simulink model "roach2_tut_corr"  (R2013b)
settings: Solver=VariableStepDiscrete  SolverMode=SingleTasking  StartTime=0.0  StopTime=100  RelTol=1e-3
undefined symbols (not defined in the file): add_latency, addr_width, Bit, bitfield, BitWidth, bram_latency, burst_size, casper_library_scopes, conv_latency, data_width, DelayLen, fan_latency, FFTSize, FFTStage, getfield, increment, led, Location, Lower, mult_latency, mux_latency, n_bits, n_bits_data, n_inputs, n_streams, n_taps, neg_latency, negate_latency, nsamples, pfb_size, pulse_len, reset_period, ROACH, ROACH2, snapshot, sx475t, sync_period, sync_period_bits, Upper, UseCounter, Width
libraries: xbsIndex_r4 x24444, casper_library_misc x73, xbsReplacements_r4 x34, casper_library_delays x14, xps_library x7
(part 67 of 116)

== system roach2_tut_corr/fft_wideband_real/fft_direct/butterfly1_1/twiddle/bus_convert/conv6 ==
  note: (ones_bit & 1) -> round-to-even (ones_bit ^ 1) -> round-to-odd (sign_bit & 1)-> round-to-zero (sign_bit ^ 1) -> round-to-inf (X ~| 1) -> round half down (X | 1) -> round half up
  in : Inport
  Concat : xbsIndex_r4/Concat  num_inputs=2  dbl_ovrd=off  block_type=concat
  Constant : xbsIndex_r4/Constant  const=1  gui_display_data_type=Fixed-point  arith_type=Unsigned  n_bits=1  bin_pt=0  preci_type=Single  exp_width=8  frac_width=24  explicit_period=off  period=1  equ=P=C  opselect=C  inp2=PCIN>>17  opr=+  inp1=P  carry=CIN  dbl_ovrd=off  block_type=constant
  Reinterpret : xbsIndex_r4/Reinterpret  force_arith_type=on  arith_type=Unsigned  force_bin_pt=on  bin_pt=0  block_type=reinterpret
  adder : xbsIndex_r4/AddSub  mode=Addition  use_carryin=off  use_carryout=off  en=off  latency=1  precision=User Defined  arith_type="Signed  (2's comp)"  n_bits=19  bin_pt=17  quantization=Truncate  overflow=Wrap  dbl_ovrd=off  use_behavioral_HDL=off  hw_selection=Fabric  pipelined=on  use_rpm=on  block_type=addsub
  almost_half : xbsIndex_r4/Constant  const=131071  gui_display_data_type=Fixed-point  arith_type=Unsigned  n_bits=35  bin_pt=0  preci_type=Single  exp_width=8  frac_width=24  explicit_period=off  period=1  equ=P=C  opselect=C  inp2=PCIN>>17  opr=+  inp1=P  carry=CIN  dbl_ovrd=off  block_type=constant
  bit : xbsIndex_r4/Slice  nbits=1  boolean_output=off  mode=Lower Bit Location + Width  bit1=0  base1=MSB of Input  bit0=17  base0=LSB of Input  dbl_ovrd=off  block_type=slice
  force1 : xbsIndex_r4/Reinterpret  force_arith_type=on  arith_type="Signed  (2's comp)"  force_bin_pt=on  bin_pt=35  block_type=reinterpret
  force2 : xbsIndex_r4/Reinterpret  force_arith_type=off  arith_type="Signed  (2's comp)"  force_bin_pt=on  bin_pt=35  block_type=reinterpret
  tweak_op : xbsIndex_r4/Logical  logical_function=AND  inputs=2  en=off  latency=0  precision=Full  arith_type=Unsigned  n_bits=8  bin_pt=2  align_bp=on  dbl_ovrd=off  block_type=logical
  out : Outport
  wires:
  tweak_op/1 -> Concat/2
  Constant/1 -> tweak_op/2
  bit/1 -> tweak_op/1
  almost_half/1 -> force2/1
  in/1 -> Reinterpret/1, bit/1
  Concat/1 -> force1/1
  Reinterpret/1 -> Concat/1
  force1/1 -> adder/1
  force2/1 -> adder/2
  adder/1 -> out/1

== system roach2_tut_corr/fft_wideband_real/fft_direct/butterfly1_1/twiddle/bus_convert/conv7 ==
  note: (ones_bit & 1) -> round-to-even (ones_bit ^ 1) -> round-to-odd (sign_bit & 1)-> round-to-zero (sign_bit ^ 1) -> round-to-inf (X ~| 1) -> round half down (X | 1) -> round half up
  in : Inport
  Concat : xbsIndex_r4/Concat  num_inputs=2  dbl_ovrd=off  block_type=concat
  Constant : xbsIndex_r4/Constant  const=1  gui_display_data_type=Fixed-point  arith_type=Unsigned  n_bits=1  bin_pt=0  preci_type=Single  exp_width=8  frac_width=24  explicit_period=off  period=1  equ=P=C  opselect=C  inp2=PCIN>>17  opr=+  inp1=P  carry=CIN  dbl_ovrd=off  block_type=constant
  Reinterpret : xbsIndex_r4/Reinterpret  force_arith_type=on  arith_type=Unsigned  force_bin_pt=on  bin_pt=0  block_type=reinterpret
  adder : xbsIndex_r4/AddSub  mode=Addition  use_carryin=off  use_carryout=off  en=off  latency=1  precision=User Defined  arith_type="Signed  (2's comp)"  n_bits=19  bin_pt=17  quantization=Truncate  overflow=Wrap  dbl_ovrd=off  use_behavioral_HDL=off  hw_selection=Fabric  pipelined=on  use_rpm=on  block_type=addsub
  almost_half : xbsIndex_r4/Constant  const=131071  gui_display_data_type=Fixed-point  arith_type=Unsigned  n_bits=35  bin_pt=0  preci_type=Single  exp_width=8  frac_width=24  explicit_period=off  period=1  equ=P=C  opselect=C  inp2=PCIN>>17  opr=+  inp1=P  carry=CIN  dbl_ovrd=off  block_type=constant
  bit : xbsIndex_r4/Slice  nbits=1  boolean_output=off  mode=Lower Bit Location + Width  bit1=0  base1=MSB of Input  bit0=17  base0=LSB of Input  dbl_ovrd=off  block_type=slice
  force1 : xbsIndex_r4/Reinterpret  force_arith_type=on  arith_type="Signed  (2's comp)"  force_bin_pt=on  bin_pt=35  block_type=reinterpret
  force2 : xbsIndex_r4/Reinterpret  force_arith_type=off  arith_type="Signed  (2's comp)"  force_bin_pt=on  bin_pt=35  block_type=reinterpret
  tweak_op : xbsIndex_r4/Logical  logical_function=AND  inputs=2  en=off  latency=0  precision=Full  arith_type=Unsigned  n_bits=8  bin_pt=2  align_bp=on  dbl_ovrd=off  block_type=logical
  out : Outport
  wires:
  tweak_op/1 -> Concat/2
  Constant/1 -> tweak_op/2
  bit/1 -> tweak_op/1
  almost_half/1 -> force2/1
  in/1 -> Reinterpret/1, bit/1
  Concat/1 -> force1/1
  Reinterpret/1 -> Concat/1
  force1/1 -> adder/1
  force2/1 -> adder/2
  adder/1 -> out/1

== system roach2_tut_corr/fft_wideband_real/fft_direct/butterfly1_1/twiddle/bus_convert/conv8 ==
  note: (ones_bit & 1) -> round-to-even (ones_bit ^ 1) -> round-to-odd (sign_bit & 1)-> round-to-zero (sign_bit ^ 1) -> round-to-inf (X ~| 1) -> round half down (X | 1) -> round half up
  in : Inport
  Concat : xbsIndex_r4/Concat  num_inputs=2  dbl_ovrd=off  block_type=concat
  Constant : xbsIndex_r4/Constant  const=1  gui_display_data_type=Fixed-point  arith_type=Unsigned  n_bits=1  bin_pt=0  preci_type=Single  exp_width=8  frac_width=24  explicit_period=off  period=1  equ=P=C  opselect=C  inp2=PCIN>>17  opr=+  inp1=P  carry=CIN  dbl_ovrd=off  block_type=constant
  Reinterpret : xbsIndex_r4/Reinterpret  force_arith_type=on  arith_type=Unsigned  force_bin_pt=on  bin_pt=0  block_type=reinterpret
  adder : xbsIndex_r4/AddSub  mode=Addition  use_carryin=off  use_carryout=off  en=off  latency=1  precision=User Defined  arith_type="Signed  (2's comp)"  n_bits=19  bin_pt=17  quantization=Truncate  overflow=Wrap  dbl_ovrd=off  use_behavioral_HDL=off  hw_selection=Fabric  pipelined=on  use_rpm=on  block_type=addsub
  almost_half : xbsIndex_r4/Constant  const=131071  gui_display_data_type=Fixed-point  arith_type=Unsigned  n_bits=35  bin_pt=0  preci_type=Single  exp_width=8  frac_width=24  explicit_period=off  period=1  equ=P=C  opselect=C  inp2=PCIN>>17  opr=+  inp1=P  carry=CIN  dbl_ovrd=off  block_type=constant
  bit : xbsIndex_r4/Slice  nbits=1  boolean_output=off  mode=Lower Bit Location + Width  bit1=0  base1=MSB of Input  bit0=17  base0=LSB of Input  dbl_ovrd=off  block_type=slice
  force1 : xbsIndex_r4/Reinterpret  force_arith_type=on  arith_type="Signed  (2's comp)"  force_bin_pt=on  bin_pt=35  block_type=reinterpret
  force2 : xbsIndex_r4/Reinterpret  force_arith_type=off  arith_type="Signed  (2's comp)"  force_bin_pt=on  bin_pt=35  block_type=reinterpret
  tweak_op : xbsIndex_r4/Logical  logical_function=AND  inputs=2  en=off  latency=0  precision=Full  arith_type=Unsigned  n_bits=8  bin_pt=2  align_bp=on  dbl_ovrd=off  block_type=logical
  out : Outport
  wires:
  tweak_op/1 -> Concat/2
  Constant/1 -> tweak_op/2
  bit/1 -> tweak_op/1
  almost_half/1 -> force2/1
  in/1 -> Reinterpret/1, bit/1
  Concat/1 -> force1/1
  Reinterpret/1 -> Concat/1
  force1/1 -> adder/1
  force2/1 -> adder/2
  adder/1 -> out/1

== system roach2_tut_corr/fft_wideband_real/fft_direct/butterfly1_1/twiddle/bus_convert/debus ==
  bus_in : Inport
  reinterpret{1..8} (8 alike) : xbsIndex_r4/Reinterpret  force_arith_type=on  arith_type="Signed  (2's comp)"  force_bin_pt=on  bin_pt=34  block_type=reinterpret
  slice1 : xbsIndex_r4/Slice  nbits=37  boolean_output=off  mode=Upper Bit Location + Width  bit1=-259  base1=MSB of Input  bit0=0  base0=LSB of Input  dbl_ovrd=off  block_type=slice
  slice2 : xbsIndex_r4/Slice  nbits=37  boolean_output=off  mode=Upper Bit Location + Width  bit1=-222  base1=MSB of Input  bit0=0  base0=LSB of Input  dbl_ovrd=off  block_type=slice
  slice3 : xbsIndex_r4/Slice  nbits=37  boolean_output=off  mode=Upper Bit Location + Width  bit1=-185  base1=MSB of Input  bit0=0  base0=LSB of Input  dbl_ovrd=off  block_type=slice
  slice4 : xbsIndex_r4/Slice  nbits=37  boolean_output=off  mode=Upper Bit Location + Width  bit1=-148  base1=MSB of Input  bit0=0  base0=LSB of Input  dbl_ovrd=off  block_type=slice
  slice5 : xbsIndex_r4/Slice  nbits=37  boolean_output=off  mode=Upper Bit Location + Width  bit1=-111  base1=MSB of Input  bit0=0  base0=LSB of Input  dbl_ovrd=off  block_type=slice
  slice6 : xbsIndex_r4/Slice  nbits=37  boolean_output=off  mode=Upper Bit Location + Width  bit1=-74  base1=MSB of Input  bit0=0  base0=LSB of Input  dbl_ovrd=off  block_type=slice
  slice7 : xbsIndex_r4/Slice  nbits=37  boolean_output=off  mode=Upper Bit Location + Width  bit1=-37  base1=MSB of Input  bit0=0  base0=LSB of Input  dbl_ovrd=off  block_type=slice
  slice8 : xbsIndex_r4/Slice  nbits=37  boolean_output=off  mode=Upper Bit Location + Width  bit1=0  base1=MSB of Input  bit0=0  base0=LSB of Input  dbl_ovrd=off  block_type=slice
  msb_out8 : Outport
  out7 : Outport  Port=2
  out6 : Outport  Port=3
  out5 : Outport  Port=4
  out4 : Outport  Port=5
  out3 : Outport  Port=6
  out2 : Outport  Port=7
  lsb_out1 : Outport  Port=8
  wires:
  bus_in/1 -> slice8/1, slice7/1, slice6/1, slice5/1, slice4/1, slice3/1, slice2/1, slice1/1
  slice8/1 -> reinterpret8/1
  reinterpret8/1 -> msb_out8/1
  slice7/1 -> reinterpret7/1
  reinterpret7/1 -> out7/1
  slice6/1 -> reinterpret6/1
  reinterpret6/1 -> out6/1
  slice5/1 -> reinterpret5/1
  reinterpret5/1 -> out5/1
  slice4/1 -> reinterpret4/1
  reinterpret4/1 -> out4/1
  slice3/1 -> reinterpret3/1
  reinterpret3/1 -> out3/1
  slice2/1 -> reinterpret2/1
  reinterpret2/1 -> out2/1
  slice1/1 -> reinterpret1/1
  reinterpret1/1 -> lsb_out1/1

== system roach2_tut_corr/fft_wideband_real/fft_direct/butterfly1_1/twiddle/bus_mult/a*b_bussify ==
  in1 : Inport
  in2 : Inport  Port=2
  in3 : Inport  Port=3
  in4 : Inport  Port=4
  concatenate : xbsIndex_r4/Concat  num_inputs=4  dbl_ovrd=off  block_type=concat
  reinterpret{1..4} (4 alike) : xbsIndex_r4/Reinterpret  force_arith_type=on  arith_type=Unsigned  force_bin_pt=on  bin_pt=0  block_type=reinterpret
  bus_out : Outport
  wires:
  concatenate/1 -> bus_out/1
  in1/1 -> reinterpret1/1
  reinterpret1/1 -> concatenate/1
  in2/1 -> reinterpret2/1
  reinterpret2/1 -> concatenate/2
  in3/1 -> reinterpret3/1
  reinterpret3/1 -> concatenate/3
  in4/1 -> reinterpret4/1
  reinterpret4/1 -> concatenate/4

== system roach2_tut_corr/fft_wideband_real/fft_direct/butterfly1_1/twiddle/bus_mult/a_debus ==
  bus_in : Inport
  reinterpret1 : xbsIndex_r4/Reinterpret  force_arith_type=on  arith_type=Unsigned  force_bin_pt=on  bin_pt=0  block_type=reinterpret
  slice1 : xbsIndex_r4/Slice  nbits=36  boolean_output=off  mode=Upper Bit Location + Width  bit1=0  base1=MSB of Input  bit0=0  base0=LSB of Input  dbl_ovrd=off  block_type=slice
  msb_lsb_out1 : Outport
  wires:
  bus_in/1 -> slice1/1
  slice1/1 -> reinterpret1/1
  reinterpret1/1 -> msb_lsb_out1/1

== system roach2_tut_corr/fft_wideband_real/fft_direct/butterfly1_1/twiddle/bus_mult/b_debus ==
  bus_in : Inport
  reinterpret{1..4} (4 alike) : xbsIndex_r4/Reinterpret  force_arith_type=on  arith_type=Unsigned  force_bin_pt=on  bin_pt=0  block_type=reinterpret
  slice1 : xbsIndex_r4/Slice  nbits=36  boolean_output=off  mode=Upper Bit Location + Width  bit1=-108  base1=MSB of Input  bit0=0  base0=LSB of Input  dbl_ovrd=off  block_type=slice
  slice2 : xbsIndex_r4/Slice  nbits=36  boolean_output=off  mode=Upper Bit Location + Width  bit1=-72  base1=MSB of Input  bit0=0  base0=LSB of Input  dbl_ovrd=off  block_type=slice
  slice3 : xbsIndex_r4/Slice  nbits=36  boolean_output=off  mode=Upper Bit Location + Width  bit1=-36  base1=MSB of Input  bit0=0  base0=LSB of Input  dbl_ovrd=off  block_type=slice
  slice4 : xbsIndex_r4/Slice  nbits=36  boolean_output=off  mode=Upper Bit Location + Width  bit1=0  base1=MSB of Input  bit0=0  base0=LSB of Input  dbl_ovrd=off  block_type=slice
  msb_out4 : Outport
  out3 : Outport  Port=2
  out2 : Outport  Port=3
  lsb_out1 : Outport  Port=4
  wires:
  bus_in/1 -> slice4/1, slice3/1, slice2/1, slice1/1
  slice4/1 -> reinterpret4/1
  reinterpret4/1 -> msb_out4/1
  slice3/1 -> reinterpret3/1
  reinterpret3/1 -> out3/1
  slice2/1 -> reinterpret2/1
  reinterpret2/1 -> out2/1
  slice1/1 -> reinterpret1/1
  reinterpret1/1 -> lsb_out1/1

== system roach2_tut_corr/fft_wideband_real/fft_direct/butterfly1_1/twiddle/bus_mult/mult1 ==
  a : Inport
  b : Inport  Port=2
  a_expand : Subsystem  AncestorBlock=casper_library_flow_control/bus_expand
  a_replicate : Subsystem  AncestorBlock=casper_library_bus/bus_replicate
  addsub_im : xbsIndex_r4/AddSub  mode=Addition  use_carryin=off  use_carryout=off  en=off  latency=1  precision=Full  arith_type=Unsigned  n_bits=16  bin_pt=14  quantization=Truncate  overflow=Wrap  dbl_ovrd=off  use_behavioral_HDL=on  hw_selection=Fabric  pipelined=on  use_rpm=on  block_type=addsub
  addsub_re : xbsIndex_r4/AddSub  mode=Subtraction  use_carryin=off  use_carryout=off  en=off  latency=1  precision=Full  arith_type=Unsigned  n_bits=16  bin_pt=14  quantization=Truncate  overflow=Wrap  dbl_ovrd=off  use_behavioral_HDL=on  hw_selection=Fabric  pipelined=on  use_rpm=on  block_type=addsub
  b_expand : Subsystem  AncestorBlock=casper_library_flow_control/bus_expand
  b_replicate : Subsystem  AncestorBlock=casper_library_bus/bus_replicate
  convert_im : xbsIndex_r4/Convert  gui_display_data_type=Fixed-point  arith_type="Signed  (2's comp)"  n_bits=37  bin_pt=34  float_type=Single  exp_bits=8  fraction_bits=24  quantization=Truncate  overflow=Wrap  en=off  latency=0  dbl_ovrd=off  pipeline=on  block_type=convert
  convert_re : xbsIndex_r4/Convert  gui_display_data_type=Fixed-point  arith_type="Signed  (2's comp)"  n_bits=37  bin_pt=34  float_type=Single  exp_bits=8  fraction_bits=24  quantization=Truncate  overflow=Wrap  en=off  latency=0  dbl_ovrd=off  pipeline=on  block_type=convert
  imim : xbsIndex_r4/Mult  precision=Full  arith_type="Signed  (2's comp)"  n_bits=16  bin_pt=14  quantization=Truncate  overflow=Wrap  en=off  latency=3  dbl_ovrd=off  use_behavioral_HDL=on  opt=Speed  use_embedded=off  optimum_pipeline=off  pipeline=on  use_rpm=on  placement_style=Triangular  block_type=mult
  imre : xbsIndex_r4/Mult  precision=Full  arith_type="Signed  (2's comp)"  n_bits=16  bin_pt=14  quantization=Truncate  overflow=Wrap  en=off  latency=3  dbl_ovrd=off  use_behavioral_HDL=on  opt=Speed  use_embedded=off  optimum_pipeline=off  pipeline=on  use_rpm=on  placement_style=Triangular  block_type=mult
  reim : xbsIndex_r4/Mult  precision=Full  arith_type="Signed  (2's comp)"  n_bits=16  bin_pt=14  quantization=Truncate  overflow=Wrap  en=off  latency=3  dbl_ovrd=off  use_behavioral_HDL=on  opt=Speed  use_embedded=off  optimum_pipeline=off  pipeline=on  use_rpm=on  placement_style=Triangular  block_type=mult
  rere : xbsIndex_r4/Mult  precision=Full  arith_type="Signed  (2's comp)"  n_bits=16  bin_pt=14  quantization=Truncate  overflow=Wrap  en=off  latency=3  dbl_ovrd=off  use_behavioral_HDL=on  opt=Speed  use_embedded=off  optimum_pipeline=off  pipeline=on  use_rpm=on  placement_style=Triangular  block_type=mult
  ri_to_c : casper_library_misc/ri_to_c
  ab : Outport
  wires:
  a/1 -> a_replicate/1(in)
  b/1 -> b_replicate/1(in)
  a_replicate/1(out) -> a_expand/1(bus_in)
  b_replicate/1(out) -> b_expand/1(bus_in)
  a_expand/1(msb_out4) -> rere/1
  b_expand/1(msb_out4) -> rere/2
  a_expand/2(out3) -> imim/1
  b_expand/2(out3) -> imim/2
  a_expand/4(lsb_out1) -> imre/1
  b_expand/3(out2) -> imre/2
  a_expand/3(out2) -> reim/1
  b_expand/4(lsb_out1) -> reim/2
  rere/1 -> addsub_re/1
  imim/1 -> addsub_re/2
  imre/1 -> addsub_im/1
  reim/1 -> addsub_im/2
  addsub_re/1 -> convert_re/1
  addsub_im/1 -> convert_im/1
  convert_re/1 -> ri_to_c/1
  convert_im/1 -> ri_to_c/2
  ri_to_c/1 -> ab/1

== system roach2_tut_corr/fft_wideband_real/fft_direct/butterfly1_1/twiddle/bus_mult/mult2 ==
  a : Inport
  b : Inport  Port=2
  a_expand : Subsystem  AncestorBlock=casper_library_flow_control/bus_expand
  a_replicate : Subsystem  AncestorBlock=casper_library_bus/bus_replicate
  addsub_im : xbsIndex_r4/AddSub  mode=Addition  use_carryin=off  use_carryout=off  en=off  latency=1  precision=Full  arith_type=Unsigned  n_bits=16  bin_pt=14  quantization=Truncate  overflow=Wrap  dbl_ovrd=off  use_behavioral_HDL=on  hw_selection=Fabric  pipelined=on  use_rpm=on  block_type=addsub
  addsub_re : xbsIndex_r4/AddSub  mode=Subtraction  use_carryin=off  use_carryout=off  en=off  latency=1  precision=Full  arith_type=Unsigned  n_bits=16  bin_pt=14  quantization=Truncate  overflow=Wrap  dbl_ovrd=off  use_behavioral_HDL=on  hw_selection=Fabric  pipelined=on  use_rpm=on  block_type=addsub
  b_expand : Subsystem  AncestorBlock=casper_library_flow_control/bus_expand
  b_replicate : Subsystem  AncestorBlock=casper_library_bus/bus_replicate
  convert_im : xbsIndex_r4/Convert  gui_display_data_type=Fixed-point  arith_type="Signed  (2's comp)"  n_bits=37  bin_pt=34  float_type=Single  exp_bits=8  fraction_bits=24  quantization=Truncate  overflow=Wrap  en=off  latency=0  dbl_ovrd=off  pipeline=on  block_type=convert
  convert_re : xbsIndex_r4/Convert  gui_display_data_type=Fixed-point  arith_type="Signed  (2's comp)"  n_bits=37  bin_pt=34  float_type=Single  exp_bits=8  fraction_bits=24  quantization=Truncate  overflow=Wrap  en=off  latency=0  dbl_ovrd=off  pipeline=on  block_type=convert
  imim : xbsIndex_r4/Mult  precision=Full  arith_type="Signed  (2's comp)"  n_bits=16  bin_pt=14  quantization=Truncate  overflow=Wrap  en=off  latency=3  dbl_ovrd=off  use_behavioral_HDL=on  opt=Speed  use_embedded=off  optimum_pipeline=off  pipeline=on  use_rpm=on  placement_style=Triangular  block_type=mult
  imre : xbsIndex_r4/Mult  precision=Full  arith_type="Signed  (2's comp)"  n_bits=16  bin_pt=14  quantization=Truncate  overflow=Wrap  en=off  latency=3  dbl_ovrd=off  use_behavioral_HDL=on  opt=Speed  use_embedded=off  optimum_pipeline=off  pipeline=on  use_rpm=on  placement_style=Triangular  block_type=mult
  reim : xbsIndex_r4/Mult  precision=Full  arith_type="Signed  (2's comp)"  n_bits=16  bin_pt=14  quantization=Truncate  overflow=Wrap  en=off  latency=3  dbl_ovrd=off  use_behavioral_HDL=on  opt=Speed  use_embedded=off  optimum_pipeline=off  pipeline=on  use_rpm=on  placement_style=Triangular  block_type=mult
  rere : xbsIndex_r4/Mult  precision=Full  arith_type="Signed  (2's comp)"  n_bits=16  bin_pt=14  quantization=Truncate  overflow=Wrap  en=off  latency=3  dbl_ovrd=off  use_behavioral_HDL=on  opt=Speed  use_embedded=off  optimum_pipeline=off  pipeline=on  use_rpm=on  placement_style=Triangular  block_type=mult
  ri_to_c : casper_library_misc/ri_to_c
  ab : Outport
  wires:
  a/1 -> a_replicate/1(in)
  b/1 -> b_replicate/1(in)
  a_replicate/1(out) -> a_expand/1(bus_in)
  b_replicate/1(out) -> b_expand/1(bus_in)
  a_expand/1(msb_out4) -> rere/1
  b_expand/1(msb_out4) -> rere/2
  a_expand/2(out3) -> imim/1
  b_expand/2(out3) -> imim/2
  a_expand/4(lsb_out1) -> imre/1
  b_expand/3(out2) -> imre/2
  a_expand/3(out2) -> reim/1
  b_expand/4(lsb_out1) -> reim/2
  rere/1 -> addsub_re/1
  imim/1 -> addsub_re/2
  imre/1 -> addsub_im/1
  reim/1 -> addsub_im/2
  addsub_re/1 -> convert_re/1
  addsub_im/1 -> convert_im/1
  convert_re/1 -> ri_to_c/1
  convert_im/1 -> ri_to_c/2
  ri_to_c/1 -> ab/1

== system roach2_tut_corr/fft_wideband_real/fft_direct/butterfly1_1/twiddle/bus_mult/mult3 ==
  a : Inport
  b : Inport  Port=2
  a_expand : Subsystem  AncestorBlock=casper_library_flow_control/bus_expand
  a_replicate : Subsystem  AncestorBlock=casper_library_bus/bus_replicate
  addsub_im : xbsIndex_r4/AddSub  mode=Addition  use_carryin=off  use_carryout=off  en=off  latency=1  precision=Full  arith_type=Unsigned  n_bits=16  bin_pt=14  quantization=Truncate  overflow=Wrap  dbl_ovrd=off  use_behavioral_HDL=on  hw_selection=Fabric  pipelined=on  use_rpm=on  block_type=addsub
  addsub_re : xbsIndex_r4/AddSub  mode=Subtraction  use_carryin=off  use_carryout=off  en=off  latency=1  precision=Full  arith_type=Unsigned  n_bits=16  bin_pt=14  quantization=Truncate  overflow=Wrap  dbl_ovrd=off  use_behavioral_HDL=on  hw_selection=Fabric  pipelined=on  use_rpm=on  block_type=addsub
  b_expand : Subsystem  AncestorBlock=casper_library_flow_control/bus_expand
  b_replicate : Subsystem  AncestorBlock=casper_library_bus/bus_replicate
  convert_im : xbsIndex_r4/Convert  gui_display_data_type=Fixed-point  arith_type="Signed  (2's comp)"  n_bits=37  bin_pt=34  float_type=Single  exp_bits=8  fraction_bits=24  quantization=Truncate  overflow=Wrap  en=off  latency=0  dbl_ovrd=off  pipeline=on  block_type=convert
  convert_re : xbsIndex_r4/Convert  gui_display_data_type=Fixed-point  arith_type="Signed  (2's comp)"  n_bits=37  bin_pt=34  float_type=Single  exp_bits=8  fraction_bits=24  quantization=Truncate  overflow=Wrap  en=off  latency=0  dbl_ovrd=off  pipeline=on  block_type=convert
  imim : xbsIndex_r4/Mult  precision=Full  arith_type="Signed  (2's comp)"  n_bits=16  bin_pt=14  quantization=Truncate  overflow=Wrap  en=off  latency=3  dbl_ovrd=off  use_behavioral_HDL=on  opt=Speed  use_embedded=off  optimum_pipeline=off  pipeline=on  use_rpm=on  placement_style=Triangular  block_type=mult
  imre : xbsIndex_r4/Mult  precision=Full  arith_type="Signed  (2's comp)"  n_bits=16  bin_pt=14  quantization=Truncate  overflow=Wrap  en=off  latency=3  dbl_ovrd=off  use_behavioral_HDL=on  opt=Speed  use_embedded=off  optimum_pipeline=off  pipeline=on  use_rpm=on  placement_style=Triangular  block_type=mult
  reim : xbsIndex_r4/Mult  precision=Full  arith_type="Signed  (2's comp)"  n_bits=16  bin_pt=14  quantization=Truncate  overflow=Wrap  en=off  latency=3  dbl_ovrd=off  use_behavioral_HDL=on  opt=Speed  use_embedded=off  optimum_pipeline=off  pipeline=on  use_rpm=on  placement_style=Triangular  block_type=mult
  rere : xbsIndex_r4/Mult  precision=Full  arith_type="Signed  (2's comp)"  n_bits=16  bin_pt=14  quantization=Truncate  overflow=Wrap  en=off  latency=3  dbl_ovrd=off  use_behavioral_HDL=on  opt=Speed  use_embedded=off  optimum_pipeline=off  pipeline=on  use_rpm=on  placement_style=Triangular  block_type=mult
  ri_to_c : casper_library_misc/ri_to_c
  ab : Outport
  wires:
  a/1 -> a_replicate/1(in)
  b/1 -> b_replicate/1(in)
  a_replicate/1(out) -> a_expand/1(bus_in)
  b_replicate/1(out) -> b_expand/1(bus_in)
  a_expand/1(msb_out4) -> rere/1
  b_expand/1(msb_out4) -> rere/2
  a_expand/2(out3) -> imim/1
  b_expand/2(out3) -> imim/2
  a_expand/4(lsb_out1) -> imre/1
  b_expand/3(out2) -> imre/2
  a_expand/3(out2) -> reim/1
  b_expand/4(lsb_out1) -> reim/2
  rere/1 -> addsub_re/1
  imim/1 -> addsub_re/2
  imre/1 -> addsub_im/1
  reim/1 -> addsub_im/2
  addsub_re/1 -> convert_re/1
  addsub_im/1 -> convert_im/1
  convert_re/1 -> ri_to_c/1
  convert_im/1 -> ri_to_c/2
  ri_to_c/1 -> ab/1

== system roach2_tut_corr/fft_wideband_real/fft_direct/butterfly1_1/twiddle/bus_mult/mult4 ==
  a : Inport
  b : Inport  Port=2
  a_expand : Subsystem  AncestorBlock=casper_library_flow_control/bus_expand
  a_replicate : Subsystem  AncestorBlock=casper_library_bus/bus_replicate
  addsub_im : xbsIndex_r4/AddSub  mode=Addition  use_carryin=off  use_carryout=off  en=off  latency=1  precision=Full  arith_type=Unsigned  n_bits=16  bin_pt=14  quantization=Truncate  overflow=Wrap  dbl_ovrd=off  use_behavioral_HDL=on  hw_selection=Fabric  pipelined=on  use_rpm=on  block_type=addsub
  addsub_re : xbsIndex_r4/AddSub  mode=Subtraction  use_carryin=off  use_carryout=off  en=off  latency=1  precision=Full  arith_type=Unsigned  n_bits=16  bin_pt=14  quantization=Truncate  overflow=Wrap  dbl_ovrd=off  use_behavioral_HDL=on  hw_selection=Fabric  pipelined=on  use_rpm=on  block_type=addsub
  b_expand : Subsystem  AncestorBlock=casper_library_flow_control/bus_expand
  b_replicate : Subsystem  AncestorBlock=casper_library_bus/bus_replicate
  convert_im : xbsIndex_r4/Convert  gui_display_data_type=Fixed-point  arith_type="Signed  (2's comp)"  n_bits=37  bin_pt=34  float_type=Single  exp_bits=8  fraction_bits=24  quantization=Truncate  overflow=Wrap  en=off  latency=0  dbl_ovrd=off  pipeline=on  block_type=convert
  convert_re : xbsIndex_r4/Convert  gui_display_data_type=Fixed-point  arith_type="Signed  (2's comp)"  n_bits=37  bin_pt=34  float_type=Single  exp_bits=8  fraction_bits=24  quantization=Truncate  overflow=Wrap  en=off  latency=0  dbl_ovrd=off  pipeline=on  block_type=convert
  imim : xbsIndex_r4/Mult  precision=Full  arith_type="Signed  (2's comp)"  n_bits=16  bin_pt=14  quantization=Truncate  overflow=Wrap  en=off  latency=3  dbl_ovrd=off  use_behavioral_HDL=on  opt=Speed  use_embedded=off  optimum_pipeline=off  pipeline=on  use_rpm=on  placement_style=Triangular  block_type=mult
  imre : xbsIndex_r4/Mult  precision=Full  arith_type="Signed  (2's comp)"  n_bits=16  bin_pt=14  quantization=Truncate  overflow=Wrap  en=off  latency=3  dbl_ovrd=off  use_behavioral_HDL=on  opt=Speed  use_embedded=off  optimum_pipeline=off  pipeline=on  use_rpm=on  placement_style=Triangular  block_type=mult
  reim : xbsIndex_r4/Mult  precision=Full  arith_type="Signed  (2's comp)"  n_bits=16  bin_pt=14  quantization=Truncate  overflow=Wrap  en=off  latency=3  dbl_ovrd=off  use_behavioral_HDL=on  opt=Speed  use_embedded=off  optimum_pipeline=off  pipeline=on  use_rpm=on  placement_style=Triangular  block_type=mult
  rere : xbsIndex_r4/Mult  precision=Full  arith_type="Signed  (2's comp)"  n_bits=16  bin_pt=14  quantization=Truncate  overflow=Wrap  en=off  latency=3  dbl_ovrd=off  use_behavioral_HDL=on  opt=Speed  use_embedded=off  optimum_pipeline=off  pipeline=on  use_rpm=on  placement_style=Triangular  block_type=mult
  ri_to_c : casper_library_misc/ri_to_c
  ab : Outport
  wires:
  a/1 -> a_replicate/1(in)
  b/1 -> b_replicate/1(in)
  a_replicate/1(out) -> a_expand/1(bus_in)
  b_replicate/1(out) -> b_expand/1(bus_in)
  a_expand/1(msb_out4) -> rere/1
  b_expand/1(msb_out4) -> rere/2
  a_expand/2(out3) -> imim/1
  b_expand/2(out3) -> imim/2
  a_expand/4(lsb_out1) -> imre/1
  b_expand/3(out2) -> imre/2
  a_expand/3(out2) -> reim/1
  b_expand/4(lsb_out1) -> reim/2
  rere/1 -> addsub_re/1
  imim/1 -> addsub_re/2
  imre/1 -> addsub_im/1
  reim/1 -> addsub_im/2
  addsub_re/1 -> convert_re/1
  addsub_im/1 -> convert_im/1
  convert_re/1 -> ri_to_c/1
  convert_im/1 -> ri_to_c/2
  ri_to_c/1 -> ab/1

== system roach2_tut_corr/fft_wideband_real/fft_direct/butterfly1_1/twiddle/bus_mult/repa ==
  in : Inport
  bussify : Subsystem  AncestorBlock=casper_library_flow_control/bus_create
  din0_0 : xbsIndex_r4/Delay  rst=off  infoeditControl=Selection of Reset will increase slice count due to use of real FFs and instead of SRLs  en=off  latency=1  dbl_ovrd=off  reg_retiming=on  block_type=delay
  din1_0 : xbsIndex_r4/Delay  rst=off  infoeditControl=Selection of Reset will increase slice count due to use of real FFs and instead of SRLs  en=off  latency=1  dbl_ovrd=off  reg_retiming=off  block_type=delay
  out : Outport
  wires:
  in/1 -> din0_0/1
  din0_0/1 -> din1_0/1
  din1_0/1 -> bussify/1(in1)
  bussify/1(bus_out) -> out/1

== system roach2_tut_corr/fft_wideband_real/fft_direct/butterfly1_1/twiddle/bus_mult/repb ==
  in : Inport
  bussify : Subsystem  AncestorBlock=casper_library_flow_control/bus_create
  din0_0 : xbsIndex_r4/Delay  rst=off  infoeditControl=Selection of Reset will increase slice count due to use of real FFs and instead of SRLs  en=off  latency=1  dbl_ovrd=off  reg_retiming=on  block_type=delay
  din1_0 : xbsIndex_r4/Delay  rst=off  infoeditControl=Selection of Reset will increase slice count due to use of real FFs and instead of SRLs  en=off  latency=1  dbl_ovrd=off  reg_retiming=off  block_type=delay
  out : Outport
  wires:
  in/1 -> din0_0/1
  din0_0/1 -> din1_0/1
  din1_0/1 -> bussify/1(in1)
  bussify/1(bus_out) -> out/1

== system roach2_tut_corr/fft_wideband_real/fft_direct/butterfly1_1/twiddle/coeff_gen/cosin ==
  theta : Inport
  misci : Inport  Port=2
  Constant4 : xbsIndex_r4/Constant  const=0  gui_display_data_type=Fixed-point  arith_type=Unsigned  n_bits=1  bin_pt=0  preci_type=Single  exp_width=8  frac_width=24  explicit_period=on  period=1  equ=P=C  opselect=C  inp2=PCIN>>17  opr=+  inp1=P  carry=CIN  dbl_ovrd=off  block_type=constant
  Constant5 : xbsIndex_r4/Constant  const=0  gui_display_data_type=Fixed-point  arith_type=Unsigned  n_bits=1  bin_pt=0  preci_type=Single  exp_width=8  frac_width=24  explicit_period=on  period=1  equ=P=C  opselect=C  inp2=PCIN>>17  opr=+  inp1=P  carry=CIN  dbl_ovrd=off  block_type=constant
  Delay : xbsIndex_r4/Delay  rst=off  infoeditControl=Selection of Reset will increase slice count due to use of real FFs and instead of SRLs  en=off  latency=bram_latency  dbl_ovrd=off  reg_retiming=on  block_type=delay
  Delay10 : xbsIndex_r4/Delay  rst=off  infoeditControl=Selection of Reset will increase slice count due to use of real FFs and instead of SRLs  en=off  latency=bram_latency  dbl_ovrd=off  reg_retiming=on  block_type=delay
  Delay8 : xbsIndex_r4/Delay  rst=off  infoeditControl=Selection of Reset will increase slice count due to use of real FFs and instead of SRLs  en=off  latency=bram_latency  dbl_ovrd=off  reg_retiming=on  block_type=delay
  ROM : xbsIndex_r4/ROM  depth=2^(9)  initVector=[131072 68614225921 68508844034 68403462150 68298080266 68192436239 68087054358 67981672478 67876290599 67770908722 67665526846 67560144971 67455025241 67349643368 67244261497 67138879627 67033759902 66928378034 66822996168 66717876447 66612756727 66507374864 66402255146 66297135430 66192015715 66086896001 65981776289 65876656577 65771536867 65666679302 65561559595 65456702032 65351844471 65246986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  distributed_mem=Block RAM  rst=off  init_reg=0  en=off  latency=bram_latency  gui_display_data_type=Fixed-point  arith_type=Unsigned  n_bits=n_bits*2  bin_pt=0  preci_type=Single  exp_width=8  frac_width=24  dbl_ovrd=off  optimize=Speed  use_rpm=on  block_type=sprom
  Terminator : Terminator
  Terminator1 : Terminator
  Terminator4 : Terminator
  add_convert0 : Subsystem
  add_convert1 : Subsystem
  assert : xbsIndex_r4/Assert  assert_type=on  type_source=Explicitly  gui_display_data_type=Fixed-point  arith_type=Unsigned  n_bits=9  bin_pt=0  preci_type=Single  exp_width=8  frac_width=24  assert_rate=off  rate_source=Explicitly  period=1  output_port=on  block_type=assert
  c_to_ri : casper_library_misc/c_to_ri  n_bits=n_bits  bin_pt=bin_pt
  invert0 : Subsystem
  invert1 : Subsystem
  -sin : Outport
  -cos : Outport  Port=2
  misco : Outport  Port=3
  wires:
  theta/1 -> assert/1
  assert/1 -> add_convert0/1(theta), add_convert1/1(theta)
  Constant4/1 -> add_convert0/2(misci)
  add_convert0/3(misco) -> Terminator/1
  misci/1 -> add_convert1/2(misci)
  add_convert1/3(misco) -> Delay/1
  add_convert0/2(add) -> ROM/1
  add_convert1/2(add) -> Terminator4/1
  ROM/1 -> c_to_ri/1
  add_convert1/1(negate) -> Delay8/1
  add_convert0/1(negate) -> Delay10/1
  Delay10/1 -> invert0/1(negate)
  Constant5/1 -> invert0/3(misci)
  c_to_ri/1 -> invert0/2(in)
  Delay8/1 -> invert1/1(negate)
  c_to_ri/2 -> invert1/2(in)
  invert0/2(misco) -> Terminator1/1
  Delay/1 -> invert1/3(misci)
  invert0/1(out) -> -sin/1
  invert1/1(out) -> -cos/1
  invert1/2(misco) -> misco/1

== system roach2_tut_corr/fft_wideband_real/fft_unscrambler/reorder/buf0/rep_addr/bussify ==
  in1 : Inport
  in2 : Inport  Port=2
  in3 : Inport  Port=3
  in4 : Inport  Port=4
  concatenate : xbsIndex_r4/Concat  num_inputs=4  dbl_ovrd=off  block_type=concat
  reinterpret{1..4} (4 alike) : xbsIndex_r4/Reinterpret  force_arith_type=on  arith_type=Unsigned  force_bin_pt=on  bin_pt=0  block_type=reinterpret
  bus_out : Outport
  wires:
  concatenate/1 -> bus_out/1
  in1/1 -> reinterpret1/1
  reinterpret1/1 -> concatenate/1
  in2/1 -> reinterpret2/1
  reinterpret2/1 -> concatenate/2
  in3/1 -> reinterpret3/1
  reinterpret3/1 -> concatenate/3
  in4/1 -> reinterpret4/1
  reinterpret4/1 -> concatenate/4

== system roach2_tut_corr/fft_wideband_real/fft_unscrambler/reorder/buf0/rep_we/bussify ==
  in1 : Inport
  in2 : Inport  Port=2
  in3 : Inport  Port=3
  in4 : Inport  Port=4
  concatenate : xbsIndex_r4/Concat  num_inputs=4  dbl_ovrd=off  block_type=concat
  reinterpret{1..4} (4 alike) : xbsIndex_r4/Reinterpret  force_arith_type=on  arith_type=Unsigned  force_bin_pt=on  bin_pt=0  block_type=reinterpret
  bus_out : Outport
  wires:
  concatenate/1 -> bus_out/1
  in1/1 -> reinterpret1/1
  reinterpret1/1 -> concatenate/1
  in2/1 -> reinterpret2/1
  reinterpret2/1 -> concatenate/2
  in3/1 -> reinterpret3/1
  reinterpret3/1 -> concatenate/3
  in4/1 -> reinterpret4/1
  reinterpret4/1 -> concatenate/4

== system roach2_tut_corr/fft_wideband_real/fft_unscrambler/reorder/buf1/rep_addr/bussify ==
  in1 : Inport
  in2 : Inport  Port=2
  in3 : Inport  Port=3
  in4 : Inport  Port=4
  concatenate : xbsIndex_r4/Concat  num_inputs=4  dbl_ovrd=off  block_type=concat
  reinterpret{1..4} (4 alike) : xbsIndex_r4/Reinterpret  force_arith_type=on  arith_type=Unsigned  force_bin_pt=on  bin_pt=0  block_type=reinterpret
  bus_out : Outport
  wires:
  concatenate/1 -> bus_out/1
  in1/1 -> reinterpret1/1
  reinterpret1/1 -> concatenate/1
  in2/1 -> reinterpret2/1
  reinterpret2/1 -> concatenate/2
  in3/1 -> reinterpret3/1
  reinterpret3/1 -> concatenate/3
  in4/1 -> reinterpret4/1
  reinterpret4/1 -> concatenate/4

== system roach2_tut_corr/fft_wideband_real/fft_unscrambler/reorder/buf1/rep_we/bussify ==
  in1 : Inport
  in2 : Inport  Port=2
  in3 : Inport  Port=3
  in4 : Inport  Port=4
  concatenate : xbsIndex_r4/Concat  num_inputs=4  dbl_ovrd=off  block_type=concat
  reinterpret{1..4} (4 alike) : xbsIndex_r4/Reinterpret  force_arith_type=on  arith_type=Unsigned  force_bin_pt=on  bin_pt=0  block_type=reinterpret
  bus_out : Outport
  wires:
  concatenate/1 -> bus_out/1
  in1/1 -> reinterpret1/1
  reinterpret1/1 -> concatenate/1
  in2/1 -> reinterpret2/1
  reinterpret2/1 -> concatenate/2
  in3/1 -> reinterpret3/1
  reinterpret3/1 -> concatenate/3
  in4/1 -> reinterpret4/1
  reinterpret4/1 -> concatenate/4

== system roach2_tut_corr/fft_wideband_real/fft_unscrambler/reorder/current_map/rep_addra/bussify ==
  in1 : Inport
  reinterpret1 : xbsIndex_r4/Reinterpret  force_arith_type=on  arith_type=Unsigned  force_bin_pt=on  bin_pt=0  block_type=reinterpret
  bus_out : Outport
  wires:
  in1/1 -> reinterpret1/1
  reinterpret1/1 -> bus_out/1

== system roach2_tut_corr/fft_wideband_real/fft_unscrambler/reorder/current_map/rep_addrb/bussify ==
  in1 : Inport
  reinterpret1 : xbsIndex_r4/Reinterpret  force_arith_type=on  arith_type=Unsigned  force_bin_pt=on  bin_pt=0  block_type=reinterpret
  bus_out : Outport
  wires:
  in1/1 -> reinterpret1/1
  reinterpret1/1 -> bus_out/1

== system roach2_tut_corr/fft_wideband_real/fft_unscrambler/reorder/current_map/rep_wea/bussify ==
  in1 : Inport
  reinterpret1 : xbsIndex_r4/Reinterpret  force_arith_type=on  arith_type=Unsigned  force_bin_pt=on  bin_pt=0  block_type=reinterpret
  bus_out : Outport
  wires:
  in1/1 -> reinterpret1/1
  reinterpret1/1 -> bus_out/1

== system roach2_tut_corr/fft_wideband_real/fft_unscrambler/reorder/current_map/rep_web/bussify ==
  in1 : Inport
  reinterpret1 : xbsIndex_r4/Reinterpret  force_arith_type=on  arith_type=Unsigned  force_bin_pt=on  bin_pt=0  block_type=reinterpret
  bus_out : Outport
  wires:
  in1/1 -> reinterpret1/1
  reinterpret1/1 -> bus_out/1

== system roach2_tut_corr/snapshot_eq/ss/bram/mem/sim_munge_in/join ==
  in1 : Inport
  in2 : Inport  Port=2
  concatenate : xbsIndex_r4/Concat  num_inputs=2  dbl_ovrd=off  block_type=concat
  reinterpret1 : xbsIndex_r4/Reinterpret  force_arith_type=on  arith_type=Unsigned  force_bin_pt=on  bin_pt=0  block_type=reinterpret
  reinterpret2 : xbsIndex_r4/Reinterpret  force_arith_type=on  arith_type=Unsigned  force_bin_pt=on  bin_pt=0  block_type=reinterpret
  bus_out : Outport
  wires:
  concatenate/1 -> bus_out/1
  in1/1 -> reinterpret1/1
  reinterpret1/1 -> concatenate/1
  in2/1 -> reinterpret2/1
  reinterpret2/1 -> concatenate/2

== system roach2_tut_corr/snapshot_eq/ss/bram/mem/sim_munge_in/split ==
  bus_in : Inport
  reinterpret1 : xbsIndex_r4/Reinterpret  force_arith_type=on  arith_type=Unsigned  force_bin_pt=on  bin_pt=0  block_type=reinterpret
  reinterpret2 : xbsIndex_r4/Reinterpret  force_arith_type=on  arith_type=Unsigned  force_bin_pt=on  bin_pt=0  block_type=reinterpret
  slice1 : xbsIndex_r4/Slice  nbits=32  boolean_output=off  mode=Upper Bit Location + Width  bit1=-32  base1=MSB of Input  bit0=0  base0=LSB of Input  dbl_ovrd=off  block_type=slice
  slice2 : xbsIndex_r4/Slice  nbits=32  boolean_output=off  mode=Upper Bit Location + Width  bit1=0  base1=MSB of Input  bit0=0  base0=LSB of Input  dbl_ovrd=off  block_type=slice
  msb_out2 : Outport
  lsb_out1 : Outport  Port=2
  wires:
  bus_in/1 -> slice2/1, slice1/1
  slice2/1 -> reinterpret2/1
  reinterpret2/1 -> msb_out2/1
  slice1/1 -> reinterpret1/1
  reinterpret1/1 -> lsb_out1/1

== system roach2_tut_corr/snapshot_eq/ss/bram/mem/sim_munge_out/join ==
  in1 : Inport
  in2 : Inport  Port=2
  concatenate : xbsIndex_r4/Concat  num_inputs=2  dbl_ovrd=off  block_type=concat
  reinterpret1 : xbsIndex_r4/Reinterpret  force_arith_type=on  arith_type=Unsigned  force_bin_pt=on  bin_pt=0  block_type=reinterpret
  reinterpret2 : xbsIndex_r4/Reinterpret  force_arith_type=on  arith_type=Unsigned  force_bin_pt=on  bin_pt=0  block_type=reinterpret
  bus_out : Outport
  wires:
  concatenate/1 -> bus_out/1
  in1/1 -> reinterpret1/1
  reinterpret1/1 -> concatenate/1
  in2/1 -> reinterpret2/1
  reinterpret2/1 -> concatenate/2

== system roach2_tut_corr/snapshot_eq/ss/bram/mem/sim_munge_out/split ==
  bus_in : Inport
  reinterpret1 : xbsIndex_r4/Reinterpret  force_arith_type=on  arith_type=Unsigned  force_bin_pt=on  bin_pt=0  block_type=reinterpret
  reinterpret2 : xbsIndex_r4/Reinterpret  force_arith_type=on  arith_type=Unsigned  force_bin_pt=on  bin_pt=0  block_type=reinterpret
  slice1 : xbsIndex_r4/Slice  nbits=32  boolean_output=off  mode=Upper Bit Location + Width  bit1=-32  base1=MSB of Input  bit0=0  base0=LSB of Input  dbl_ovrd=off  block_type=slice
  slice2 : xbsIndex_r4/Slice  nbits=32  boolean_output=off  mode=Upper Bit Location + Width  bit1=0  base1=MSB of Input  bit0=0  base0=LSB of Input  dbl_ovrd=off  block_type=slice
  msb_out2 : Outport
  lsb_out1 : Outport  Port=2
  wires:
  bus_in/1 -> slice2/1, slice1/1
  slice2/1 -> reinterpret2/1
  reinterpret2/1 -> msb_out2/1
  slice1/1 -> reinterpret1/1
  reinterpret1/1 -> lsb_out1/1

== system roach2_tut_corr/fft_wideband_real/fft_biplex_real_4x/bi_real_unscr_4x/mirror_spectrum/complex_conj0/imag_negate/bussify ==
  in1 : Inport
  in2 : Inport  Port=2
  in3 : Inport  Port=3
  in4 : Inport  Port=4
  concatenate : xbsIndex_r4/Concat  num_inputs=4  dbl_ovrd=off  block_type=concat
  reinterpret{1..4} (4 alike) : xbsIndex_r4/Reinterpret  force_arith_type=on  arith_type=Unsigned  force_bin_pt=on  bin_pt=0  block_type=reinterpret
  bus_out : Outport
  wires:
  concatenate/1 -> bus_out/1
  in1/1 -> reinterpret1/1
  reinterpret1/1 -> concatenate/1
  in2/1 -> reinterpret2/1
  reinterpret2/1 -> concatenate/2
  in3/1 -> reinterpret3/1
  reinterpret3/1 -> concatenate/3
  in4/1 -> reinterpret4/1
  reinterpret4/1 -> concatenate/4

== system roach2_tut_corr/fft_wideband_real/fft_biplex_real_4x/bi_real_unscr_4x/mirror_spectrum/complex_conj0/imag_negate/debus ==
  bus_in : Inport
  reinterpret{1..4} (4 alike) : xbsIndex_r4/Reinterpret  force_arith_type=on  arith_type="Signed  (2's comp)"  force_bin_pt=on  bin_pt=17  block_type=reinterpret
  slice1 : xbsIndex_r4/Slice  nbits=18  boolean_output=off  mode=Upper Bit Location + Width  bit1=-54  base1=MSB of Input  bit0=0  base0=LSB of Input  dbl_ovrd=off  block_type=slice
  slice2 : xbsIndex_r4/Slice  nbits=18  boolean_output=off  mode=Upper Bit Location + Width  bit1=-36  base1=MSB of Input  bit0=0  base0=LSB of Input  dbl_ovrd=off  block_type=slice
  slice3 : xbsIndex_r4/Slice  nbits=18  boolean_output=off  mode=Upper Bit Location + Width  bit1=-18  base1=MSB of Input  bit0=0  base0=LSB of Input  dbl_ovrd=off  block_type=slice
  slice4 : xbsIndex_r4/Slice  nbits=18  boolean_output=off  mode=Upper Bit Location + Width  bit1=0  base1=MSB of Input  bit0=0  base0=LSB of Input  dbl_ovrd=off  block_type=slice
  msb_out4 : Outport
  out3 : Outport  Port=2
  out2 : Outport  Port=3
  lsb_out1 : Outport  Port=4
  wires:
  bus_in/1 -> slice4/1, slice3/1, slice2/1, slice1/1
  slice4/1 -> reinterpret4/1
  reinterpret4/1 -> msb_out4/1
  slice3/1 -> reinterpret3/1
  reinterpret3/1 -> out3/1
  slice2/1 -> reinterpret2/1
  reinterpret2/1 -> out2/1
  slice1/1 -> reinterpret1/1
  reinterpret1/1 -> lsb_out1/1

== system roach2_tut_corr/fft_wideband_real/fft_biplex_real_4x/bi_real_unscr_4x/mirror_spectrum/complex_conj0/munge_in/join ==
  in1 : Inport
  in2 : Inport  Port=2
  in3 : Inport  Port=3
  in4 : Inport  Port=4
  in5 : Inport  Port=5
  in6 : Inport  Port=6
  in7 : Inport  Port=7
  in8 : Inport  Port=8
  concatenate : xbsIndex_r4/Concat  num_inputs=8  dbl_ovrd=off  block_type=concat
  reinterpret{1..8} (8 alike) : xbsIndex_r4/Reinterpret  force_arith_type=on  arith_type=Unsigned  force_bin_pt=on  bin_pt=0  block_type=reinterpret
  bus_out : Outport
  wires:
  concatenate/1 -> bus_out/1
  in1/1 -> reinterpret1/1
  reinterpret1/1 -> concatenate/1
  in2/1 -> reinterpret2/1
  reinterpret2/1 -> concatenate/2
  in3/1 -> reinterpret3/1
  reinterpret3/1 -> concatenate/3
  in4/1 -> reinterpret4/1
  reinterpret4/1 -> concatenate/4
  in5/1 -> reinterpret5/1
  reinterpret5/1 -> concatenate/5
  in6/1 -> reinterpret6/1
  reinterpret6/1 -> concatenate/6
  in7/1 -> reinterpret7/1
  reinterpret7/1 -> concatenate/7
  in8/1 -> reinterpret8/1
  reinterpret8/1 -> concatenate/8

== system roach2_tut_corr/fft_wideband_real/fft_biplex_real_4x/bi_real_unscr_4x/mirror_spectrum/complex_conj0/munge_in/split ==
  bus_in : Inport
  reinterpret{1..8} (8 alike) : xbsIndex_r4/Reinterpret  force_arith_type=on  arith_type=Unsigned  force_bin_pt=on  bin_pt=0  block_type=reinterpret
  slice1 : xbsIndex_r4/Slice  nbits=18  boolean_output=off  mode=Upper Bit Location + Width  bit1=-126  base1=MSB of Input  bit0=0  base0=LSB of Input  dbl_ovrd=off  block_type=slice
  slice2 : xbsIndex_r4/Slice  nbits=18  boolean_output=off  mode=Upper Bit Location + Width  bit1=-108  base1=MSB of Input  bit0=0  base0=LSB of Input  dbl_ovrd=off  block_type=slice
  slice3 : xbsIndex_r4/Slice  nbits=18  boolean_output=off  mode=Upper Bit Location + Width  bit1=-90  base1=MSB of Input  bit0=0  base0=LSB of Input  dbl_ovrd=off  block_type=slice
  slice4 : xbsIndex_r4/Slice  nbits=18  boolean_output=off  mode=Upper Bit Location + Width  bit1=-72  base1=MSB of Input  bit0=0  base0=LSB of Input  dbl_ovrd=off  block_type=slice
  slice5 : xbsIndex_r4/Slice  nbits=18  boolean_output=off  mode=Upper Bit Location + Width  bit1=-54  base1=MSB of Input  bit0=0  base0=LSB of Input  dbl_ovrd=off  block_type=slice
  slice6 : xbsIndex_r4/Slice  nbits=18  boolean_output=off  mode=Upper Bit Location + Width  bit1=-36  base1=MSB of Input  bit0=0  base0=LSB of Input  dbl_ovrd=off  block_type=slice
  slice7 : xbsIndex_r4/Slice  nbits=18  boolean_output=off  mode=Upper Bit Location + Width  bit1=-18  base1=MSB of Input  bit0=0  base0=LSB of Input  dbl_ovrd=off  block_type=slice
  slice8 : xbsIndex_r4/Slice  nbits=18  boolean_output=off  mode=Upper Bit Location + Width  bit1=0  base1=MSB of Input  bit0=0  base0=LSB of Input  dbl_ovrd=off  block_type=slice
  msb_out8 : Outport
  out7 : Outport  Port=2
  out6 : Outport  Port=3
  out5 : Outport  Port=4
  out4 : Outport  Port=5
  out3 : Outport  Port=6
  out2 : Outport  Port=7
  lsb_out1 : Outport  Port=8
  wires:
  bus_in/1 -> slice8/1, slice7/1, slice6/1, slice5/1, slice4/1, slice3/1, slice2/1, slice1/1
  slice8/1 -> reinterpret8/1
  reinterpret8/1 -> msb_out8/1
  slice7/1 -> reinterpret7/1
  reinterpret7/1 -> out7/1
  slice6/1 -> reinterpret6/1
  reinterpret6/1 -> out6/1
  slice5/1 -> reinterpret5/1
  reinterpret5/1 -> out5/1
  slice4/1 -> reinterpret4/1
  reinterpret4/1 -> out4/1
  slice3/1 -> reinterpret3/1
  reinterpret3/1 -> out3/1
  slice2/1 -> reinterpret2/1
  reinterpret2/1 -> out2/1
  slice1/1 -> reinterpret1/1
  reinterpret1/1 -> lsb_out1/1

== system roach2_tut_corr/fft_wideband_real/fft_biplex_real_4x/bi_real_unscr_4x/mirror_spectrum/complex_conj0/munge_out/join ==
  in1 : Inport
  in2 : Inport  Port=2
  in3 : Inport  Port=3
  in4 : Inport  Port=4
  in5 : Inport  Port=5
  in6 : Inport  Port=6
  in7 : Inport  Port=7
  in8 : Inport  Port=8
  concatenate : xbsIndex_r4/Concat  num_inputs=8  dbl_ovrd=off  block_type=concat
  reinterpret{1..8} (8 alike) : xbsIndex_r4/Reinterpret  force_arith_type=on  arith_type=Unsigned  force_bin_pt=on  bin_pt=0  block_type=reinterpret
  bus_out : Outport
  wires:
  concatenate/1 -> bus_out/1
  in1/1 -> reinterpret1/1
  reinterpret1/1 -> concatenate/1
  in2/1 -> reinterpret2/1
  reinterpret2/1 -> concatenate/2
  in3/1 -> reinterpret3/1
  reinterpret3/1 -> concatenate/3
  in4/1 -> reinterpret4/1
  reinterpret4/1 -> concatenate/4
  in5/1 -> reinterpret5/1
  reinterpret5/1 -> concatenate/5
  in6/1 -> reinterpret6/1
  reinterpret6/1 -> concatenate/6
  in7/1 -> reinterpret7/1
  reinterpret7/1 -> concatenate/7
  in8/1 -> reinterpret8/1
  reinterpret8/1 -> concatenate/8

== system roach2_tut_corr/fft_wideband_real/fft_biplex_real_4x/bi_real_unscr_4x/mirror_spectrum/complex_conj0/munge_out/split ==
  bus_in : Inport
  reinterpret{1..8} (8 alike) : xbsIndex_r4/Reinterpret  force_arith_type=on  arith_type=Unsigned  force_bin_pt=on  bin_pt=0  block_type=reinterpret
  slice1 : xbsIndex_r4/Slice  nbits=18  boolean_output=off  mode=Upper Bit Location + Width  bit1=-126  base1=MSB of Input  bit0=0  base0=LSB of Input  dbl_ovrd=off  block_type=slice
  slice2 : xbsIndex_r4/Slice  nbits=18  boolean_output=off  mode=Upper Bit Location + Width  bit1=-108  base1=MSB of Input  bit0=0  base0=LSB of Input  dbl_ovrd=off  block_type=slice
  slice3 : xbsIndex_r4/Slice  nbits=18  boolean_output=off  mode=Upper Bit Location + Width  bit1=-90  base1=MSB of Input  bit0=0  base0=LSB of Input  dbl_ovrd=off  block_type=slice
  slice4 : xbsIndex_r4/Slice  nbits=18  boolean_output=off  mode=Upper Bit Location + Width  bit1=-72  base1=MSB of Input  bit0=0  base0=LSB of Input  dbl_ovrd=off  block_type=slice
  slice5 : xbsIndex_r4/Slice  nbits=18  boolean_output=off  mode=Upper Bit Location + Width  bit1=-54  base1=MSB of Input  bit0=0  base0=LSB of Input  dbl_ovrd=off  block_type=slice
  slice6 : xbsIndex_r4/Slice  nbits=18  boolean_output=off  mode=Upper Bit Location + Width  bit1=-36  base1=MSB of Input  bit0=0  base0=LSB of Input  dbl_ovrd=off  block_type=slice
  slice7 : xbsIndex_r4/Slice  nbits=18  boolean_output=off  mode=Upper Bit Location + Width  bit1=-18  base1=MSB of Input  bit0=0  base0=LSB of Input  dbl_ovrd=off  block_type=slice
  slice8 : xbsIndex_r4/Slice  nbits=18  boolean_output=off  mode=Upper Bit Location + Width  bit1=0  base1=MSB of Input  bit0=0  base0=LSB of Input  dbl_ovrd=off  block_type=slice
  msb_out8 : Outport
  out7 : Outport  Port=2
  out6 : Outport  Port=3
  out5 : Outport  Port=4
  out4 : Outport  Port=5
  out3 : Outport  Port=6
  out2 : Outport  Port=7
  lsb_out1 : Outport  Port=8
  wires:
  bus_in/1 -> slice8/1, slice7/1, slice6/1, slice5/1, slice4/1, slice3/1, slice2/1, slice1/1
  slice8/1 -> reinterpret8/1
  reinterpret8/1 -> msb_out8/1
  slice7/1 -> reinterpret7/1
  reinterpret7/1 -> out7/1
  slice6/1 -> reinterpret6/1
  reinterpret6/1 -> out6/1
  slice5/1 -> reinterpret5/1
  reinterpret5/1 -> out5/1
  slice4/1 -> reinterpret4/1
  reinterpret4/1 -> out4/1
  slice3/1 -> reinterpret3/1
  reinterpret3/1 -> out3/1
  slice2/1 -> reinterpret2/1
  reinterpret2/1 -> out2/1
  slice1/1 -> reinterpret1/1
  reinterpret1/1 -> lsb_out1/1

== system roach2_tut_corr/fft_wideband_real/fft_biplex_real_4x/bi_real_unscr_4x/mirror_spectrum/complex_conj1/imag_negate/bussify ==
  in1 : Inport
  in2 : Inport  Port=2
  in3 : Inport  Port=3
  in4 : Inport  Port=4
  concatenate : xbsIndex_r4/Concat  num_inputs=4  dbl_ovrd=off  block_type=concat
  reinterpret{1..4} (4 alike) : xbsIndex_r4/Reinterpret  force_arith_type=on  arith_type=Unsigned  force_bin_pt=on  bin_pt=0  block_type=reinterpret
  bus_out : Outport
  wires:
  concatenate/1 -> bus_out/1
  in1/1 -> reinterpret1/1
  reinterpret1/1 -> concatenate/1
  in2/1 -> reinterpret2/1
  reinterpret2/1 -> concatenate/2
  in3/1 -> reinterpret3/1
  reinterpret3/1 -> concatenate/3
  in4/1 -> reinterpret4/1
  reinterpret4/1 -> concatenate/4
